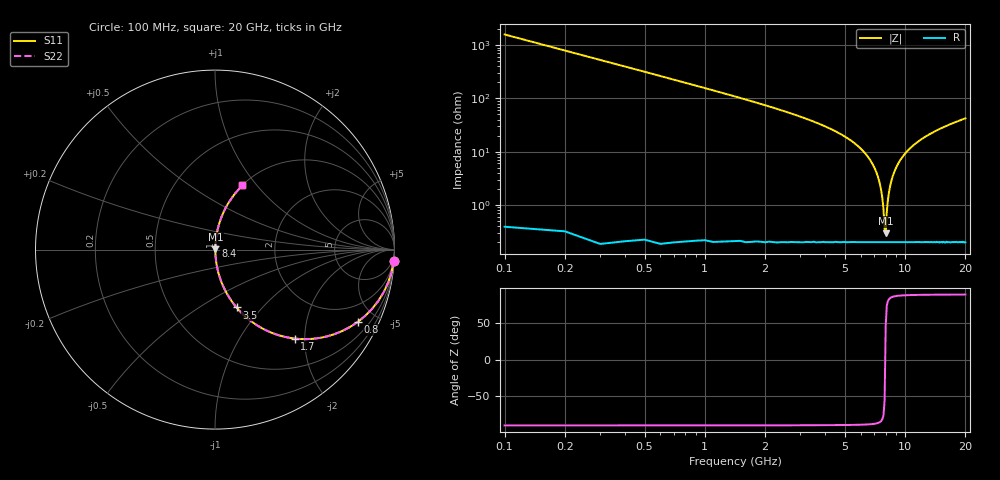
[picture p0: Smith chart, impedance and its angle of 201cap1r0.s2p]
! AVX Thin Film Operation		Date: May 2007
! Description: Accu-P® Series, Thin Film, SMD, RF Capacitor
! Part Number: 02013J1R0ABS
! 50 MHz  -  20.05 GHz
! Serial Measurements
# hz S db R 50
!	S11		S21		S12		S22
!	dB	Phase	dB	Phase	dB	Phase	dB	Phase
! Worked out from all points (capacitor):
!   200 points, 100 MHz to 20 GHz, reference 50 ohm
!   read as one part in series: C = 1 pF near 200 MHz
!   lowest |Z| = 291 mohm at 8 GHz (marker M1)
!   series resonance near 7.958 GHz, so ESL is about 400 pH
!   S11 on the Smith chart (normalised r, x): 100 MHz: 1, -32; 800 MHz: 1.00, -3.94; 1.7 GHz: 1.00, -1.79; 3.5 GHz: 1.00, -0.73; 8.4 GHz: 1.00, +0.04; 20 GHz: 1.00, +0.85
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1e8  -0.02 -3.6  -24.05 86.4  -24.05 86.4  -0.02 -3.6
2e8  -0.07 -7.2  -18.08 82.8  -18.08 82.8  -0.07 -7.2
3e8  -0.15 -10.7  -14.63 79.3  -14.63 79.3  -0.15 -10.7
5e8  -0.41 -17.5  -10.44 72.5  -10.44 72.5  -0.41 -17.5
8e8  -1.00 -26.9  -6.89 63.0  -6.89 63.0  -1.00 -26.9
1.7e9  -3.54 -48.1  -2.56 41.7  -2.56 41.7  -3.54 -48.1
3.5e9  -9.28 -69.6  -0.56 20.1  -0.56 20.1  -9.28 -69.6
5.6e9  -16.97 -81.0  -0.11 8.1  -0.11 8.1  -16.97 -81.0
6.8e9  -24.02 -84.6  -0.03 3.6  -0.03 3.6  -24.02 -84.6
7.3e9  -29.24 -84.7  -0.02 2.0  -0.02 2.0  -29.24 -84.7
7.6e9  -34.67 -82.7  -0.02 1.1  -0.02 1.1  -34.67 -82.7
7.8e9  -41.68 -75.5  -0.02 0.5  -0.02 0.5  -41.68 -75.5
7.9e9  -49.05 -55.4  -0.02 0.2  -0.02 0.2  -49.05 -55.4
8e9  -50.73 46.5  -0.02 -0.1  -0.02 -0.1  -50.73 46.5
8.1e9  -42.67 73.8  -0.02 -0.4  -0.02 -0.4  -42.67 73.8
8.2e9  -38.32 79.8  -0.02 -0.7  -0.02 -0.7  -38.32 79.8
8.4e9  -33.28 83.5  -0.02 -1.2  -0.02 -1.2  -33.28 83.5
9e9  -26.15 84.9  -0.03 -2.8  -0.03 -2.8  -26.15 84.9
1.01e10  -20.39 83.3  -0.06 -5.5  -0.06 -5.5  -20.39 83.3
1.34e10  -13.45 77.2  -0.22 -12.3  -0.22 -12.3  -13.45 77.2
1.67e10  -10.23 71.7  -0.45 -17.9  -0.45 -17.9  -10.23 71.7
2e10  -8.20 66.8  -0.73 -22.9  -0.73 -22.9  -8.20 66.8
